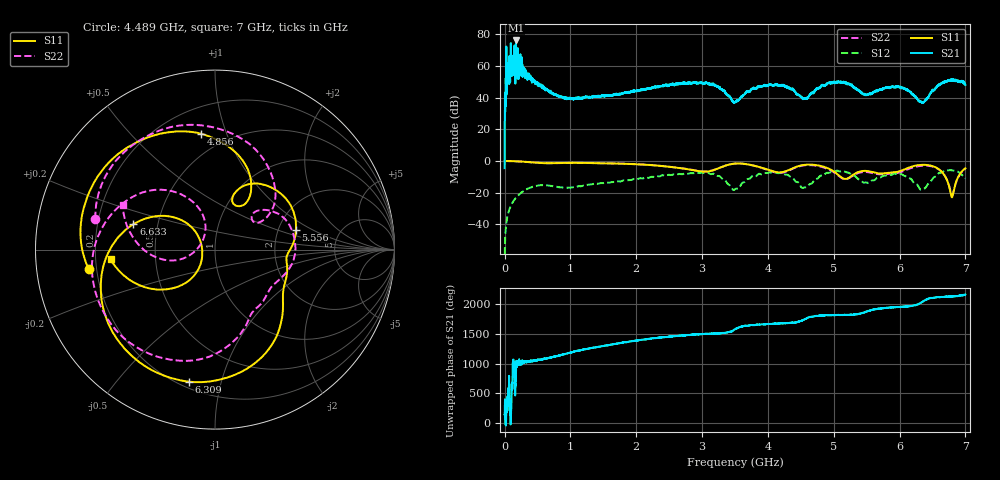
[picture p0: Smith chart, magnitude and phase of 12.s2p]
!Keysight Technologies,N5232A,MY52221221,A.10.65.11
!Date: Wednesday, October 16, 2024 12:04:16
!Correction: S11(Full 2 Port(1,4))
!S41(Full 2 Port(1,4))
!S14(Full 2 Port(1,4))
!S44(Full 2 Port(1,4))
!S2P File: Measurements: S11, S41, S14, S44:
# Hz S  RI  R 50
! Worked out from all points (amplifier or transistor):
!   4001 points, 300 kHz to 7 GHz, reference 50 ohm
!   highest |S21| = 76.2 dB at 173.5 MHz (marker M1)
!   |S21| within 3 dB of that: 94.56267 MHz to 94.93493 MHz (372.3 kHz wide, 0.393 % of centre)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
!   unconditionally stable (mu >= 1): start of sweep to 385.7 kHz
!   at 1.166 GHz: K = 6.98, MSG = 27.7 dB, |S12| = -16.0 dB
!   at 3.5 GHz: K = 4.21, MSG = 27.4 dB, |S12| = -17.9 dB
!   at 7 GHz: K = 35.28, MSG = 29.6 dB, |S12| = -11.1 dB
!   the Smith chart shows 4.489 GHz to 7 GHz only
!   S11 on the Smith chart (normalised r, x): 4.489 GHz: 0.17, -0.07; 4.856 GHz: 0.36, +0.82; 5.556 GHz: 2.51, +0.69; 6.309 GHz: 0.24, -0.79; 6.633 GHz: 0.36, +0.13; 7 GHz: 0.26, -0.04
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300000  -0.9961 -0.0108  -0.4515 0.3846  1.58e-05 2.12e-05  -0.992 -0.0153
6.32973e7  -0.9726 0.2061  -1276 462.1  0.00648 0.025  -0.9714 0.2117
1.122952e8  -0.9227 0.3588  -359.7 -1114  0.0199 0.041  -0.9182 0.3663
1.297944e8  -0.8974 0.4064  581.6 -959  0.026 0.0456  -0.8914 0.4178
1.350442e8  -0.8902 0.4213  1281 -1154  0.028 0.0468  -0.8844 0.432
1.385441e8  -0.8847 0.4309  -551.5 -1029  0.0294 0.0476  -0.8786 0.4421
1.735426e8  -0.8256 0.5246  -3747 5225  0.0445 0.0538  -0.8176 0.5376
2.155408e8  -0.7397 0.6232  253.6 -305.9  0.0649 0.0559  -0.7273 0.6378
3.27536e8  -0.4663 0.8121  269.9 -350.1  0.1214 0.0321  -0.4424 0.8256
5.37527e8  0.0672 0.8616  243.8 -71.46  0.1383 -0.101  0.1073 0.859
1.1675e9  0.8472 -0.2136  -81.78 47.19  -0.0827 -0.1357  0.8238 -0.2883
2.3347e9  -0.6373 0.3117  216.3 -21.09  0.1184 0.3052  -0.5689 0.4334
3.053919e9  0.2623 0.3789  134 260.3  0.1826 -0.3726  0.3536 0.3077
3.50015e9  0.7923 -0.2333  -53.42 44.69  -0.057 -0.1131  0.6994 -0.4397
4.488858e9  -0.7039 -0.1081  4.56 -111.9  0.0493 0.1635  -0.6674 0.171
4.66735e9  -0.6174 0.456  137.4 -35.33  -0.0489 0.1892  -0.3556 0.644
4.856342e9  -0.0787 0.646  243.4 34.05  0.0861 0.3533  0.1958 0.5854
5.556312e9  0.4511 0.1077  -4.995 135.6  0.1621 -0.1557  0.418 -0.0993
5.83455e9  0.4008 -0.1349  -159.9 127.4  0.0157 -0.3724  0.2689 -0.2862
6.30878e9  -0.1461 -0.7355  -59.63 -42.34  -0.129 -0.0159  -0.4237 -0.5516
6.632516e9  -0.4548 0.1413  220.2 -178.5  -0.4263 -0.00772  -0.3323 0.333
7e9  -0.5822 -0.053  252.6 9.533  0.0871 0.2649  -0.5136 0.2462
